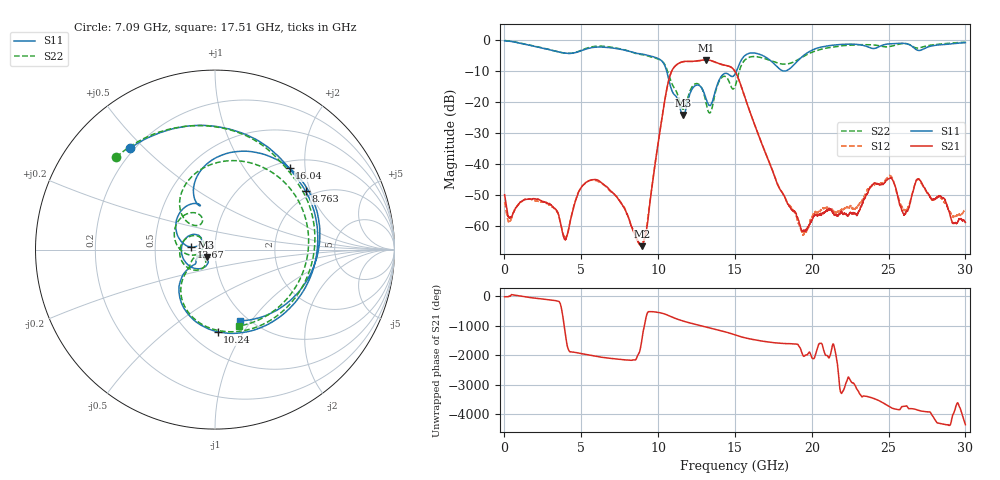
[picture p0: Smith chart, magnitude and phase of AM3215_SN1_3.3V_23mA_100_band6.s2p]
!Agilent Technologies,E8364B,MY43040894,A.07.50.67
!Agilent E8364B: A.07.50.67
!Date: Tuesday, May 25, 2021 15:27:55
!Correction: S11(Full 2 Port(1,2))
!S21(Full 2 Port(1,2))
!S12(Full 2 Port(1,2))
!S22(Full 2 Port(1,2))
!S2P File: Measurements: S11, S21, S12, S22:
# Hz S  dB  R 50
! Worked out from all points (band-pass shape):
!   6401 points, 10 MHz to 30 GHz, reference 50 ohm
!   highest |S21| = -6.43 dB at 13.1 GHz (marker M1); lowest = -66.4 dB at 8.946 GHz (marker M2)
!   |S21| within 3 dB of the highest: 10.95 GHz to 14.9 GHz (3.951 GHz wide, 30.6 % of centre)
!   lowest |S11| = -24.2 dB at 11.62 GHz (marker M3), VSWR 1.13, Z = 45.4 - j3.68 ohm
!   |S11| at or under -10 dB: 10.55 GHz to 15.11 GHz (4.551 GHz wide, 35.5 % of centre); 18.14 GHz to 18.29 GHz (147.4 MHz wide, 0.809 % of centre)
!   |S22| runs from -23.5 to -0.2 dB; largest |S21 - S12| = 0.0055
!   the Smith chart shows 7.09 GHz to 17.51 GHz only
!   S11 on the Smith chart (normalised r, x): 7.09 GHz: 0.18, +0.45; 8.763 GHz: 1.82, +1.85; 10.24 GHz: 0.67, -0.77; 13.67 GHz: 0.77, +0.02; 16.04 GHz: 1.14, +1.66; 17.51 GHz: 0.92, -0.88
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1e7  -0.33 -6.4  -49.86 -30.6  -52.20 -52.8  -0.18 -6.7
9.612453e8  -1.02 -85.4  -52.61 -0.8  -52.80 -1.2  -0.94 -84.4
2.128044e9  -2.28 -168.3  -51.35 -87.1  -51.94 -86.9  -2.18 -166.0
3.590056e9  -3.95 86.3  -57.78 140.9  -57.77 148.8  -3.95 92.6
5.009895e9  -3.47 -64.6  -47.46 -149.1  -47.38 -151.2  -3.31 -55.8
6.045488e9  -2.31 -160.5  -45.10 111.1  -45.40 110.9  -2.03 -152.9
7.090452e9  -2.64 130.1  -49.46 39.4  -49.43 40.8  -2.46 136.8
8.763331e9  -4.43 32.8  -65.44 -119.8  -65.83 -145.9  -4.59 37.0
8.946083e9  -4.55 21.0  -66.43 -26.8  -66.24 42.3  -4.73 24.9
1.000979e10  -6.02 -62.8  -32.98 162.5  -32.99 162.0  -6.16 -60.1
1.02394e10  -6.79 -88.2  -25.51 137.3  -25.53 136.8  -6.79 -84.2
1.162175e10  -24.17 -139.2  -7.02 -127.9  -7.04 -127.8  -22.33 -142.3
1.310251e10  -18.59 138.7  -6.43 32.1  -6.48 32.2  -19.86 140.4
1.366951e10  -17.49 173.9  -7.05 -43.4  -7.12 -43.3  -18.15 -165.5
1.5005e10  -11.04 111.6  -10.14 123.4  -10.24 123.3  -15.04 130.4
1.603591e10  -4.22 47.5  -24.01 -18.5  -24.00 -17.5  -5.46 56.2
1.751198e10  -7.53 -70.5  -43.01 -139.5  -42.86 -139.4  -7.01 -72.5
1.865066e10  -8.93 158.1  -54.42 -175.8  -53.96 -174.7  -7.44 -178.2
2.00049e10  -3.35 59.5  -57.97 75.6  -57.15 -11.2  -4.01 83.8
2.200579e10  -1.44 -9.9  -55.89 7.2  -54.43 152.5  -1.88 2.0
2.500479e10  -1.29 -59.1  -44.75 -128.9  -43.87 -127.7  -2.18 -60.5
3e10  -0.89 -111.7  -58.82 -27.8  -54.55 4.0  -0.75 -114.6
